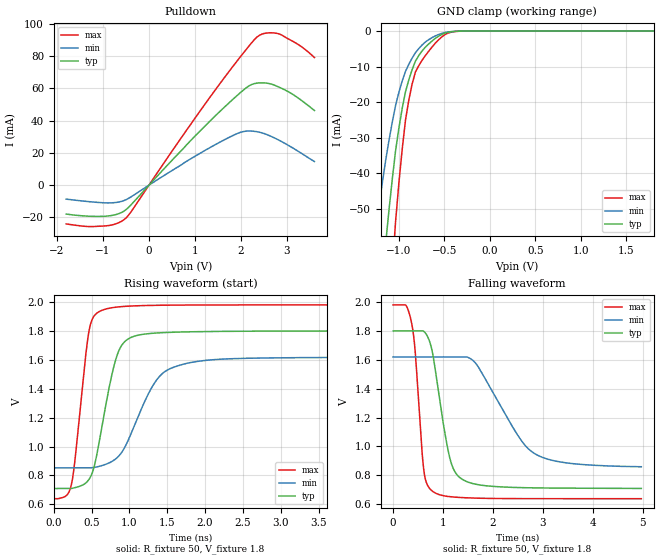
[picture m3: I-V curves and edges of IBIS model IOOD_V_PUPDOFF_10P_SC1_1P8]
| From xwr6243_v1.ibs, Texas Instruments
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|   Model Cell IOOD_V_PUPDOFF_10P_SC1_1P8
|IOOD_V_PUPDOFF_10P_SC1_1P8
[Model]   IOOD_V_PUPDOFF_10P_SC1_1P8
Model_type   I/O_open_drain
Polarity   Non-Inverting
Enable   Active-Low
Vinl =  0.63
Vinh =  1.17
Cref =  15pF
Rref =  100.0000M
Vref =  0V
Vmeas =  0.9
|   typ   min   max
C_comp   2.290246p   2.205796p   2.292736p
[Model Spec]
Vinl   0.63   0.567   0.693
Vinh   1.17   1.053   1.287
[Temperature Range]   25   125   -40
[Voltage Range]   1.8   1.62   1.98
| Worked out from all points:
|   slope of the pulldown table from 0 to 0.27 V, typ, clamps not added: 32.2 ohm
|   GND clamp passes 1 mA (typ) near -0.53 V on its own axis
|   rising waveform, R_fixture 50, V_fixture 1.8: 20-80 % time 246ps typ, 417ps min, 160ps max; typ from 0.709 V to 1.8 V
|   falling waveform, R_fixture 50, V_fixture 1.8: 20-80 % time 308ps typ, 788ps min, 165ps max; typ from 1.8 V to 0.709 V
| Where Nom  PVT is Nominal Process, 1.8V, 25C
|   Fast PVT is Strong Process,  1.98V, -40C
|   Slow PVT is Weak Process,   1.62V, 125C
[Pulldown]
|   voltage   I(typ)   I(min)   I(max)
-1.8V     -17.92mA   -8.674mA   -24.03mA
-927.3mV  -19.22mA   -10.99mA   -25.2mA
-654.5mV  -17.65mA   -10.46mA   -23.22mA
-490.9mV  -14.97mA   -8.904mA   -20.12mA
872.7mV   26.63mA    15.72mA    36.29mA
1.691V    49.7mA     28.87mA    68.59mA
2.127V    60.63mA    33.53mA    84.59mA
2.4V      63.43mA    32.84mA    92.9mA
2.618V    62.99mA    30.74mA    94.47mA
2.836V    60.69mA    27.76mA    93.76mA
3.273V    53.49mA    20.53mA    86.73mA
3.6V      46.26mA    14.64mA    79.12mA
[GND_clamp]
|   voltage   I(typ)   I(min)   I(max)
-1.8V     -270.2mA   -170.2mA   -430.1mA
-1.255V   -91.66mA   -55.91mA   -148.4mA
-1.145V   -59.91mA   -36.44mA   -97.09mA
-1.109V   -50.48mA   -30.83mA   -81.55mA
-1.073V   -41.73mA   -25.65mA   -67.05mA
-1.036V   -33.66mA   -20.92mA   -53.59mA
-927.3mV  -17.07mA   -11.35mA   -25.04mA
-854.5mV  -10.86mA   -7.616mA   -14.91mA
-781.8mV  -6.919mA   -4.945mA   -9.771mA
-636.4mV  -2.823mA   -1.868mA   -4.529mA
-381.8mV  -84.73uA   -78.7uA    -126.1uA
1.8V      19.3nA     3.129uA    310.3nA
[Ramp]
| variable   typ   min   max
dV/dt_f 0.66170168/0.31099039n 0.46782709/0.81087951n 0.81106408/0.16651847n
dV/dt_r 0.65944917/0.43266267n 0.47442459/1.0514017n 0.81583107/0.23074199n
R_load = 50
[Rising Waveform]
R_fixture = 50
V_fixture = 1.8
V_fixture_min = 1.62
V_fixture_max = 1.98
|   time   V(typ)   V(min)   V(max)
0s        709.3mV    852.1mV    638.8mV
228.2ps   709.3mV    852.1mV    728.2mV
277.2ps   715.1mV    852.1mV    895mV
458.2ps   767.3mV    852.1mV    1.778V
607.5ps   1.053V     863.6mV    1.936V
833.5ps   1.626V     920.9mV    1.965V
1.059ns   1.763V     1.136V     1.973V
1.377ns   1.786V     1.473V     1.978V
1.755ns   1.793V     1.575V     1.979V
4.974ns   1.8V       1.618V     1.98V
[Falling Waveform]
R_fixture = 50
V_fixture = 1.8
V_fixture_min = 1.62
V_fixture_max = 1.98
|   time   V(typ)   V(min)   V(max)
0s        1.8V       1.62V      1.981V
367.8ps   1.8V       1.62V      1.86V
439.5ps   1.8V       1.62V      1.67V
612.7ps   1.799V     1.62V      842.8mV
786.7ps   1.654V     1.62V      690.4mV
1.123ns   939.6mV    1.62V      652.7mV
1.375ns   774.7mV    1.62V      645.6mV
1.662ns   737.7mV    1.573V     641.7mV
2.828ns   713mV      952.2mV    638.2mV
4.974ns   709mV      859.5mV    637.9mV
